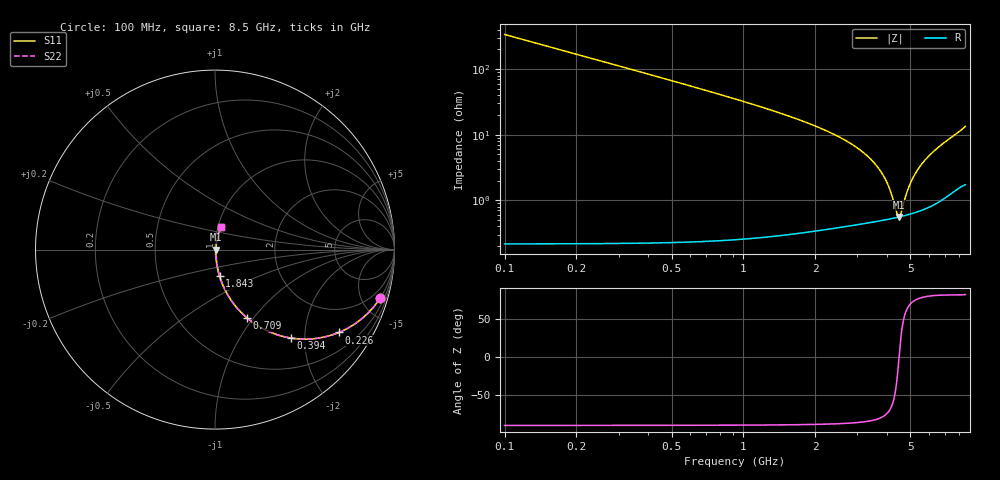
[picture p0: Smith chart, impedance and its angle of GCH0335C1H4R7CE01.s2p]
!Murata Part Number: GCH0335C1H4R7CE01
!These Parameters are Measured in Series Mode Connection
!Data Generated on Mar 13, 2026
!  o--ll--o
!Port1  Port2
!  o------o
!Operation Temp=25[degC], DC Bias Voltage=0[V]
!Freq. Start=100[MHz] Stop=9[GHz] 401[Steps]
# Hz S RI R 50
!Freq.(Hz) S11(Real) S11(Imag) S21(Real) S21(Imag) S12(Real) S12(Imag) S22(Real) S22(Imag)
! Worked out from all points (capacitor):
!   401 points, 100 MHz to 8.5 GHz, reference 50 ohm
!   read as one part in series: C = 4.7 pF near 142 MHz
!   lowest |Z| = 556 mohm at 4.489 GHz (marker M1)
!   series resonance near 4.483 GHz, so ESL is about 270 pH
!   S11 on the Smith chart (normalised r, x): 100 MHz: 1.00, -6.77; 226 MHz: 1.00, -2.99; 394 MHz: 1.00, -1.71; 709 MHz: 1.00, -0.93; 1.843 GHz: 1.01, -0.31; 8.5 GHz: 1.03, +0.27
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1e8  0.9196 -0.2716  0.0804 0.2716  0.0804 0.2716  0.9196 -0.2716
2.26e8  0.6905 -0.4616  0.3095 0.4616  0.3095 0.4616  0.6905 -0.4616
3.94e8  0.4212 -0.4925  0.5788 0.4925  0.5788 0.4925  0.4212 -0.4925
5.41e8  0.2763 -0.4453  0.7237 0.4453  0.7237 0.4453  0.2763 -0.4453
7.09e8  0.1793 -0.3811  0.8207 0.3811  0.8207 0.3811  0.1793 -0.3811
1.024e9  0.0913 -0.2839  0.9087 0.2839  0.9087 0.2839  0.0913 -0.2839
1.507e9  0.0408 -0.1905  0.9592 0.1905  0.9592 0.1905  0.0408 -0.1905
1.843e9  0.0258 -0.1482  0.9742 0.1482  0.9742 0.1482  0.0258 -0.1482
2.914e9  0.00861 -0.0665  0.9914 0.0665  0.9914 0.0665  0.00861 -0.0665
3.397e9  0.00635 -0.0424  0.9937 0.0424  0.9937 0.0424  0.00635 -0.0424
3.775e9  0.00555 -0.0262  0.9945 0.0262  0.9945 0.0262  0.00555 -0.0262
4.069e9  0.00534 -0.0148  0.9947 0.0148  0.9947 0.0148  0.00534 -0.0148
4.3e9  0.00538 -0.00637  0.9946 0.00637  0.9946 0.00637  0.00538 -0.00637
4.405e9  0.00545 -0.00269  0.9946 0.00269  0.9946 0.00269  0.00545 -0.00269
4.489e9  0.00553 0.000193  0.9945 -0.000193  0.9945 -0.000193  0.00553 0.000193
4.573e9  0.00563 0.00303  0.9944 -0.00303  0.9944 -0.00303  0.00563 0.00303
4.846e9  0.00607 0.012  0.9939 -0.012  0.9939 -0.012  0.00607 0.012
5.035e9  0.00648 0.018  0.9935 -0.018  0.9935 -0.018  0.00648 0.018
5.329e9  0.0073 0.027  0.9927 -0.027  0.9927 -0.027  0.0073 0.027
5.707e9  0.00867 0.0382  0.9913 -0.0382  0.9913 -0.0382  0.00867 0.0382
7.114e9  0.0174 0.0783  0.9826 -0.0783  0.9826 -0.0783  0.0174 0.0783
8.5e9  0.0336 0.1269  0.9664 -0.1269  0.9664 -0.1269  0.0336 0.1269
